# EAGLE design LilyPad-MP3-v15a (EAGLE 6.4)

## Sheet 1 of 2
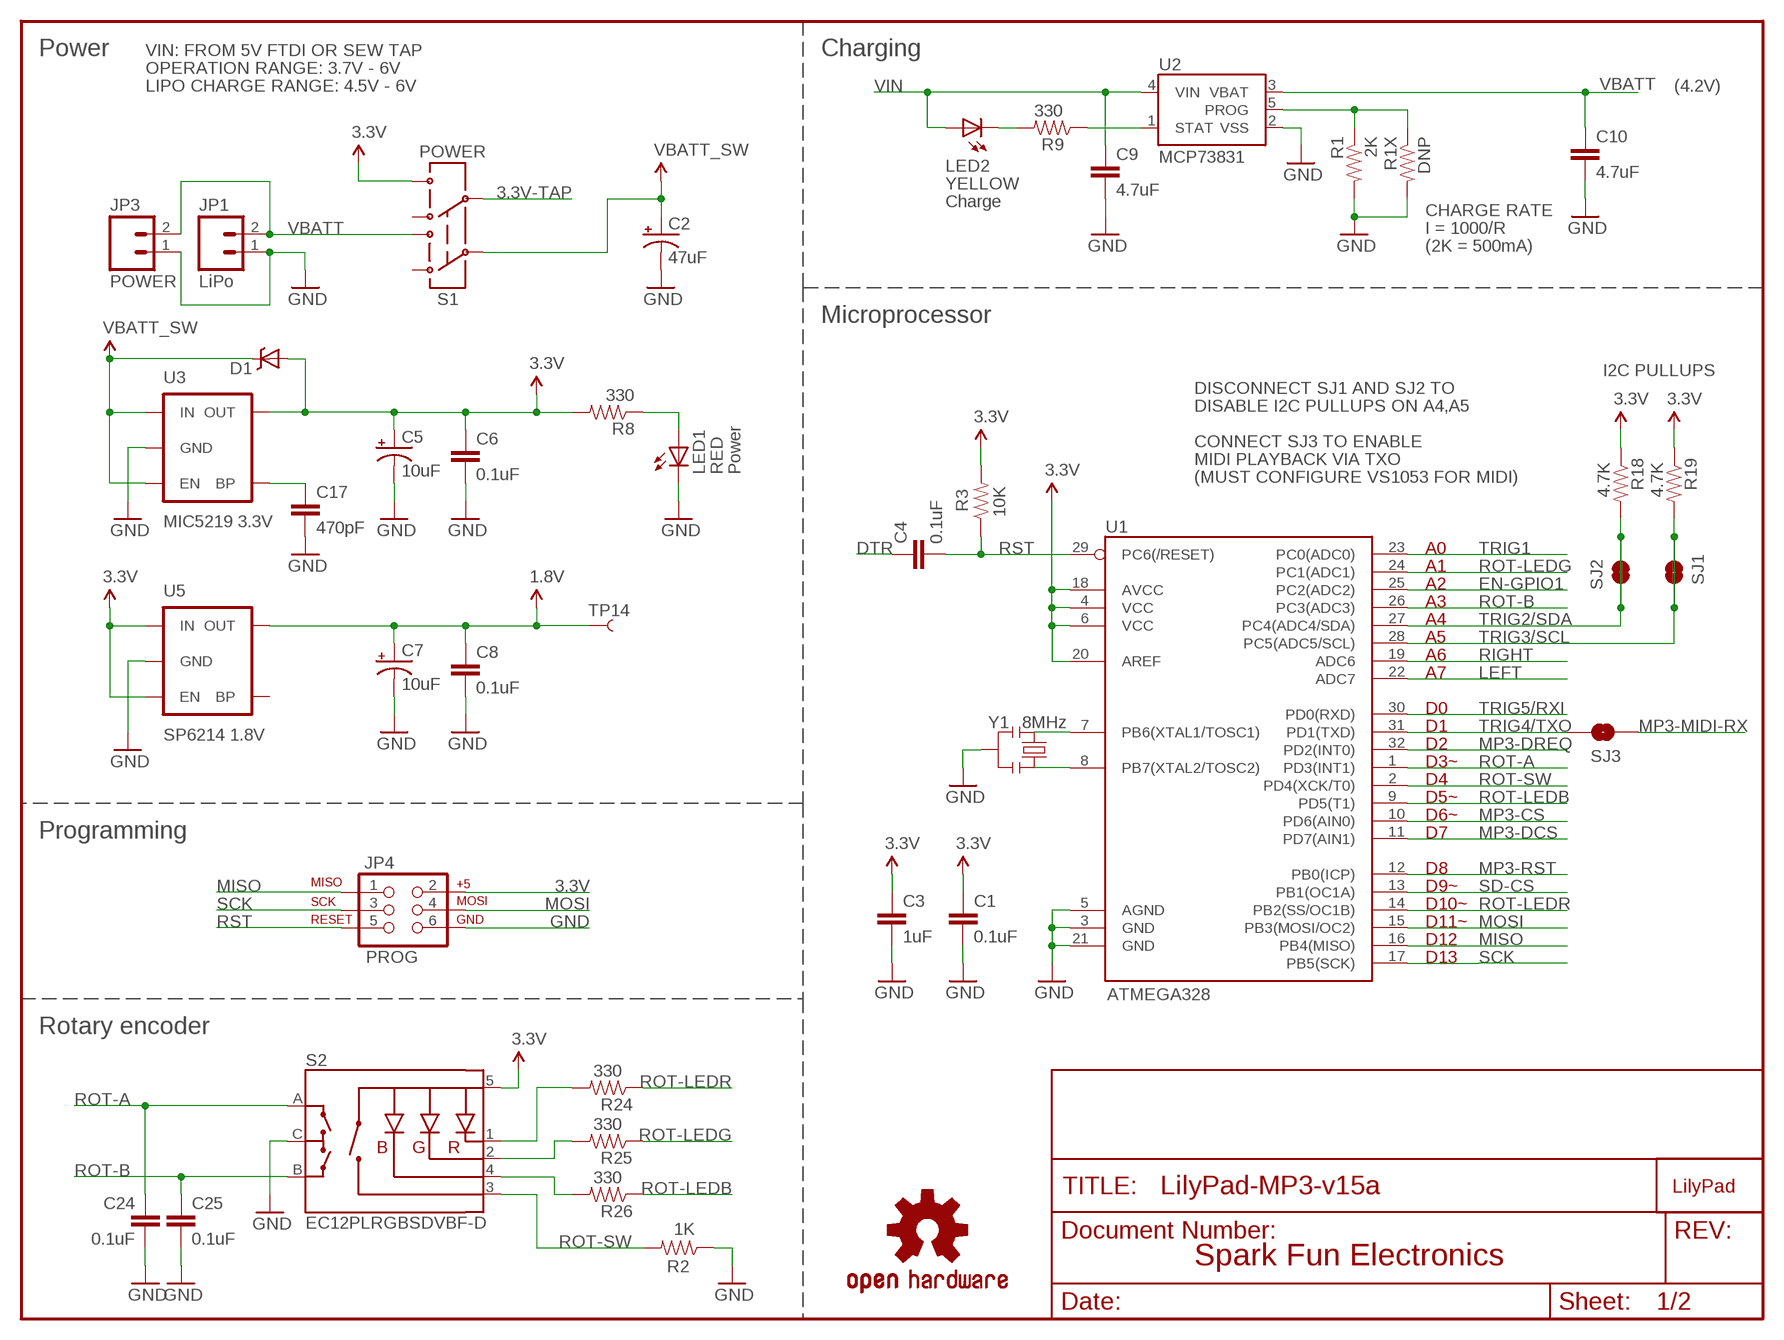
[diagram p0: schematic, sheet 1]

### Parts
C1  0.1uF  CAP0402-CAP  [0402-CAP]
C2  47uF  CAP_POL3528  [EIA3528]
C3  1uF  CAP0402-CAP  [0402-CAP]
C4  0.1uF  CAP0402-CAP  [0402-CAP]
C5  10uF  CAP_POL1206  [EIA3216]
C6  0.1uF  CAP0402-CAP  [0402-CAP]
C7  10uF  CAP_POL1206  [EIA3216]
C8  0.1uF  CAP0402-CAP  [0402-CAP]
C9  4.7uF  CAP0402-CAP  [0402-CAP]
C10  4.7uF  CAP0402-CAP  [0402-CAP]
C17  470pF  CAP0402-CAP  [0402-CAP]
C24  0.1uF  CAP0402-CAP  [0402-CAP]
C25  0.1uF  CAP0402-CAP  [0402-CAP]
D1  DIODE-SCHOTTKY  [SOD-523]
JP1  LiPo  M02-JST-2MM-SMT  [JST-2-SMD]
JP3  POWER  M02PTH  [1X02]
JP4  PROG  AVR_SPI_PRG_6NS  [2X3-NS]
LED1  RED  LED0603  [LED-0603]
LED2  YELLOW  LED0603  [LED-0603]
R1  2K  RESISTOR0402-RES  [0402-RES]
R1X  DNP  RESISTORAXIAL-0.3  [AXIAL-0.3]
R2  1K  RESISTOR0402-RES  [0402-RES]
R3  10K  RESISTOR0402-RES  [0402-RES]
R8  330  RESISTOR0402-RES  [0402-RES]
R9  330  RESISTOR0402-RES  [0402-RES]
R18  4.7K  RESISTOR0402-RES  [0402-RES]
R19  4.7K  RESISTOR0402-RES  [0402-RES]
R24  330  RESISTOR0402-RES  [0402-RES]
R25  330  RESISTOR0402-RES  [0402-RES]
R26  330  RESISTOR0402-RES  [0402-RES]
S1  POWER  AYZ0202  [AYZ0202]
S2  EC12PLRGBSDVBF-D  ENCODER_3LED_CA  [ENCODER_LED_3]
SJ1  SOLDERJUMPERNO  [SJ_2S-NO]
SJ2  SOLDERJUMPERNO  [SJ_2S-NO]
SJ3  SOLDERJUMPERNO  [SJ_2S-NO]
TP14  1.8V  TEST-POINT3X5  [PAD.03X.05]
U1  ATMEGA328  ATMEGA168  [TQFP32-08]
U2  MCP73831  [SOT23-5]
U3  MIC5219 3.3V  V_REG_LDOSMD  [SOT23-5]
U5  SP6214 1.8V  V_REG_LDOSMD2  [SC70]
U$1  LOGO-LPLP  [LOGO-LILYPAD]
U$4  OSHW-LOGOM  [OSHW-LOGO-M]
Y1  8MHz  RESONATORSMD  [RESONATOR-SMD]

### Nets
1.8V: C7.A(+) C8.1 TP14.P$1 U5.5(OUT) ; also sheet 2
3.3V: C1.1 C3.1 C5.A(+) C6.1 D1.A JP4.2 R3.2 R8.2 R18.1 R19.1 S1.4 S2.5(+) U1.4(VCC) U1.6(VCC) U1.18(AVCC) U1.20(AREF) U3.5(OUT) U5.1(IN) U5.3(EN) ; also sheet 2
3.3V-TAP: S1.5 ; also sheet 2
DTR: C4.1 ; also sheet 2
EN-GPIO1: U1.25(PC2(ADC2)) ; also sheet 2
GND [VCC]: C1.2 C2.C(-) C3.2 C5.C(-) C6.2 C7.C(-) C8.2 C9.2 C10.2 C17.2 C24.2 C25.2 JP1.1 JP3.1 JP4.6 LED1.C R1.2 R1X.P$2 R2.1 S2.C U1.3(GND) U1.5(AGND) U1.21(GND) U2.2(VSS) U3.2(GND) U5.2(GND) Y1.2 ; also sheet 2
LEFT: U1.22(ADC7) ; also sheet 2
MISO: JP4.1 U1.16(PB4(MISO)) ; also sheet 2
MOSI: JP4.4 U1.15(PB3(MOSI/OC2)) ; also sheet 2
MP3-CS: U1.10(PD6(AIN0)) ; also sheet 2
MP3-DCS: U1.11(PD7(AIN1)) ; also sheet 2
MP3-DREQ: U1.32(PD2(INT0)) ; also sheet 2
MP3-MIDI-RX: SJ3.1 ; also sheet 2
MP3-RST: U1.12(PB0(ICP)) ; also sheet 2
N$1: U1.7(PB6(XTAL1/TOSC1)) Y1.1
N$3: U1.8(PB7(XTAL2/TOSC2)) Y1.3
N$6: LED1.A R8.1
N$8: LED2.C R9.2
N$12: R24.2 S2.1(-R)
N$13: R25.2 S2.2(-G)
N$14: R26.2 S2.4(-B)
N$70: C17.1 U3.4(BP)
PROG: R1.1 R1X.P$1 U2.5(PROG)
RIGHT: U1.19(ADC6) ; also sheet 2
ROT-A: C24.1 S2.A U1.1(PD3(INT1))
ROT-B: C25.1 S2.B U1.26(PC3(ADC3))
ROT-LEDB: R26.1 U1.9(PD5(T1))
ROT-LEDG: R25.1 U1.24(PC1(ADC1))
ROT-LEDR: R24.1 U1.14(PB2(SS/OC1B))
ROT-SW: R2.2 S2.3(SW) U1.2(PD4(XCK/T0))
RST: C4.2 JP4.5 R3.1 U1.29(PC6(/RESET))
SCK: JP4.3 U1.17(PB5(SCK)) ; also sheet 2
SD-CS: U1.13(PB1(OC1A)) ; also sheet 2
STAT: R9.1 U2.1(STAT)
TRIG1: U1.23(PC0(ADC0)) ; also sheet 2
TRIG2/SDA: R18.2 SJ2.1 SJ2.2 U1.27(PC4(ADC4/SDA)) ; also sheet 2
TRIG3/SCL: R19.2 SJ1.1 SJ1.2 U1.28(PC5(ADC5/SCL)) ; also sheet 2
TRIG4/TXO: SJ3.2 U1.31(PD1(TXD)) ; also sheet 2
TRIG5/RXI: U1.30(PD0(RXD)) ; also sheet 2
VBATT: C10.1 JP1.2 JP3.2 S1.1 U2.3(VBAT)
VBATT_SW: C2.A(+) D1.C S1.2 U3.1(IN) U3.3(EN) ; also sheet 2
VIN: C9.1 LED2.A U2.4(VIN) ; also sheet 2
Unconnected: S1.3 S1.6 U5.4(BP)

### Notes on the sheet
- Power | VIN: FROM 5V FTDI OR SEW TAP | Charging
- OPERATION RANGE: 3.7V - 6V
- LIPO CHARGE RANGE: 4.5V - 6V | (4.2V)
- Charge
- CHARGE RATE
- I = 1000/R
- (2K = 500mA)
- Microprocessor
- I2C PULLUPS
- DISCONNECT SJ1 AND SJ2 TO
- DISABLE I2C PULLUPS ON A4,A5
- CONNECT SJ3 TO ENABLE
- MIDI PLAYBACK VIA TXO
- Power
- (MUST CONFIGURE VS1053 FOR MIDI)
- A0
- A1
- A2
- A3
- A4
- A5
- A6
- A7
- D0
- D1
- D2
- D3~
- D4
- D5~
- D6~
- Programming | D7
- D8
- D9~
- D10~
- D11~
- D12
- D13
- Rotary encoder
- Spark Fun Electronics

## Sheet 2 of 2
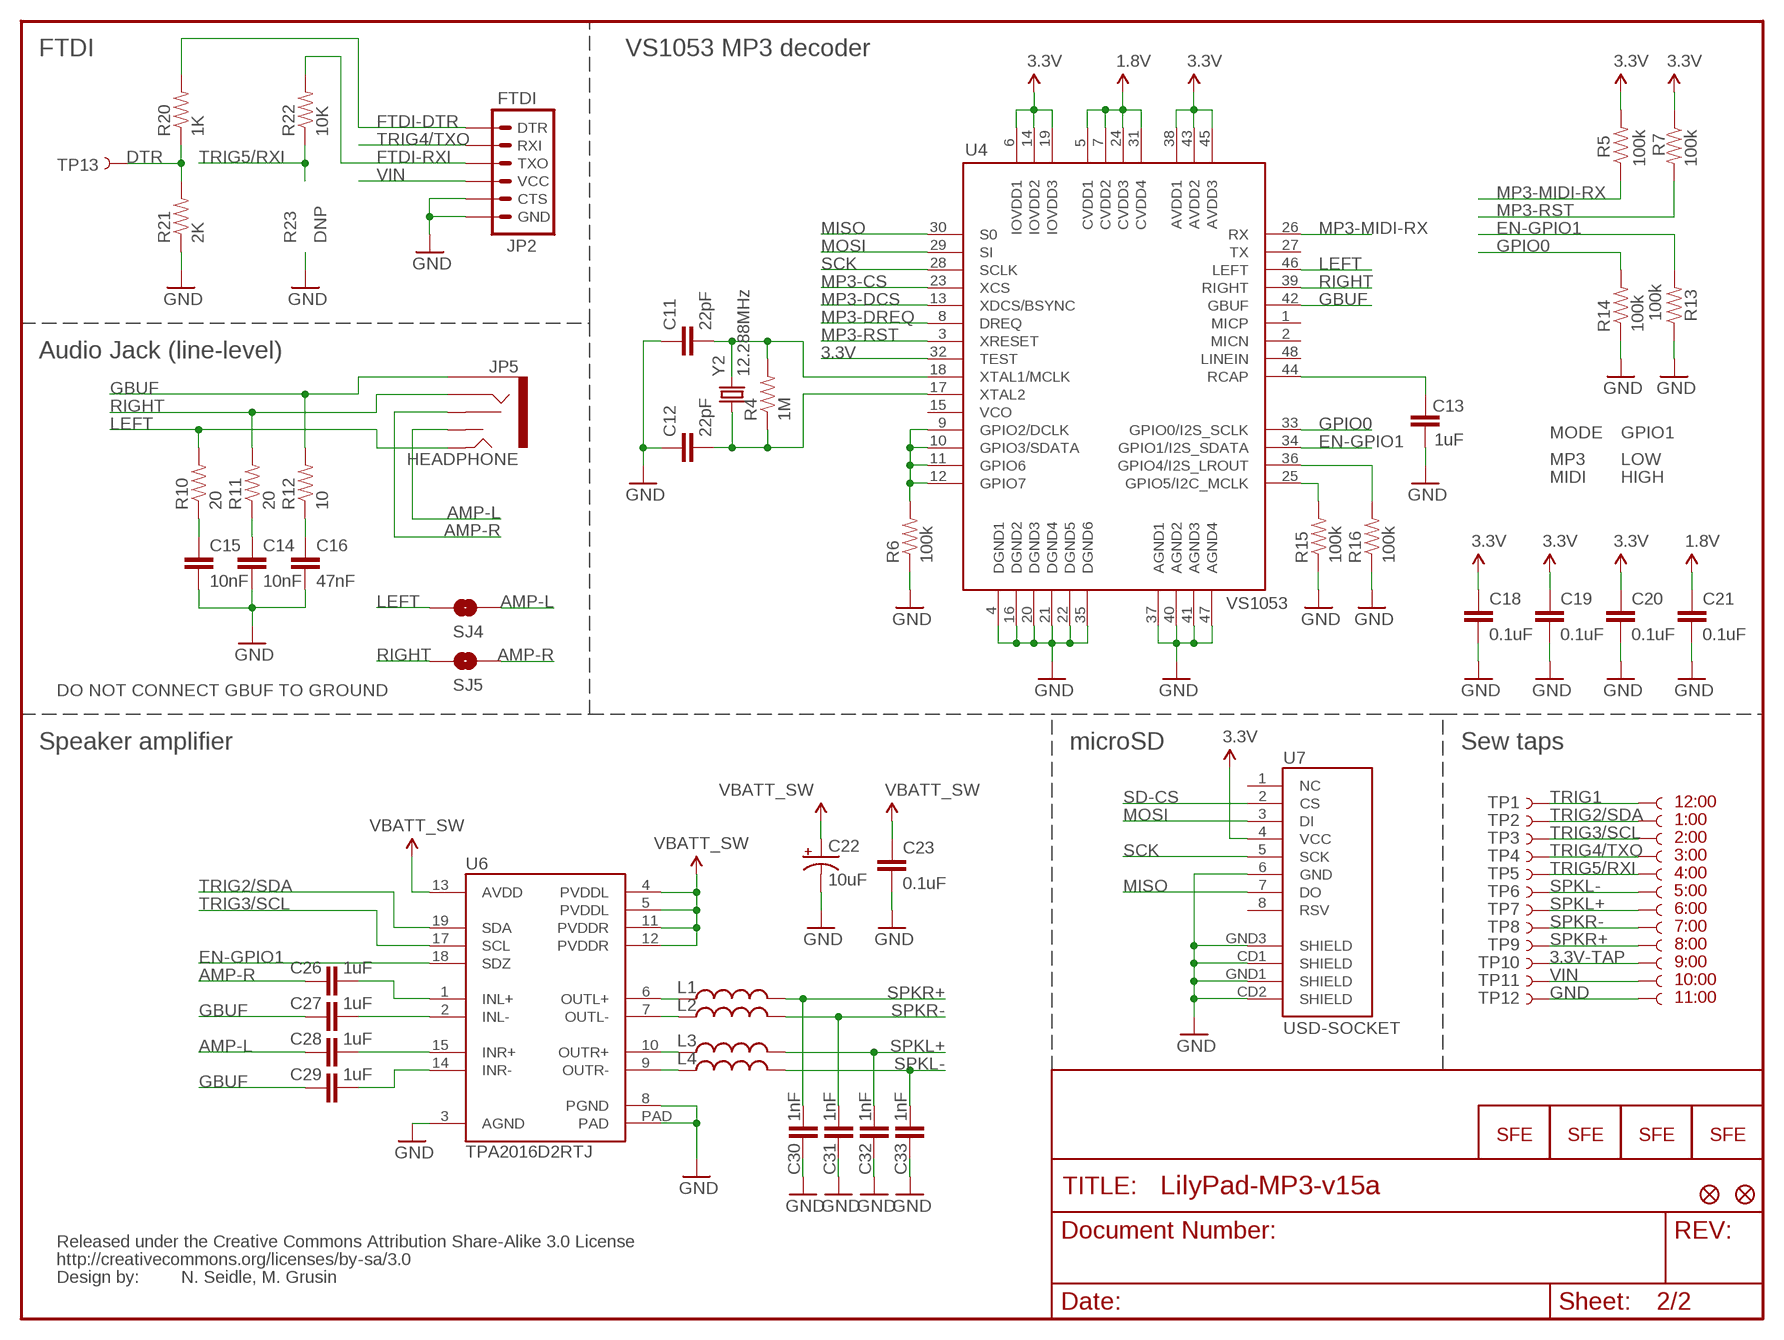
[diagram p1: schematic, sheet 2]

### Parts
C11  22pF  CAP0402-CAP  [0402-CAP]
C12  22pF  CAP0402-CAP  [0402-CAP]
C13  1uF  CAP0402-CAP  [0402-CAP]
C14  10nF  CAP0402-CAP  [0402-CAP]
C15  10nF  CAP0402-CAP  [0402-CAP]
C16  47nF  CAP0402-CAP  [0402-CAP]
C18  0.1uF  CAP0402-CAP  [0402-CAP]
C19  0.1uF  CAP0402-CAP  [0402-CAP]
C20  0.1uF  CAP0402-CAP  [0402-CAP]
C21  0.1uF  CAP0402-CAP  [0402-CAP]
C22  10uF  CAP_POL1206  [EIA3216]
C23  0.1uF  CAP0402-CAP  [0402-CAP]
C26  1uF  CAP0402-CAP  [0402-CAP]
C27  1uF  CAP0402-CAP  [0402-CAP]
C28  1uF  CAP0402-CAP  [0402-CAP]
C29  1uF  CAP0402-CAP  [0402-CAP]
C30  1nF  CAP0402-CAP  [0402-CAP]
C31  1nF  CAP0402-CAP  [0402-CAP]
C32  1nF  CAP0402-CAP  [0402-CAP]
C33  1nF  CAP0402-CAP  [0402-CAP]
JP2  FTDI  ARDUINO_SERIAL_PROGRAMSMD  [1X06-SMD]
JP5  HEADPHONE  AUDIO-JACK2SMD  [AUDIO-JACK-3.5MM-SMD]
JP6  LOGO-SFENW2  [SFE-NEW-WEB]
JP7  FIDUCIALUFIDUCIAL  [MICRO-FIDUCIAL]
JP8  FIDUCIALUFIDUCIAL  [MICRO-FIDUCIAL]
L1  INDUCTOR0805  [0805]
L2  INDUCTOR0805  [0805]
L3  INDUCTOR0805  [0805]
L4  INDUCTOR0805  [0805]
LOGO1  LOGO-SFESK  [SFE-LOGO-FLAME]
LOGO2  LOGO-SFENEW  [SFE-NEW-WEBLOGO]
LOGO3  LOGO-SFESK  [SFE-LOGO-FLAME]
R4  1M  RESISTOR0402-RES  [0402-RES]
R5  100k  RESISTOR0402-RES  [0402-RES]
R6  100k  RESISTOR0402-RES  [0402-RES]
R7  100k  RESISTOR0402-RES  [0402-RES]
R10  20  RESISTOR0402-RES  [0402-RES]
R11  20  RESISTOR0402-RES  [0402-RES]
R12  10  RESISTOR0402-RES  [0402-RES]
R13  100k  RESISTOR0402-RES  [0402-RES]
R14  100k  RESISTOR0402-RES  [0402-RES]
R15  100k  RESISTOR0402-RES  [0402-RES]
R16  100k  RESISTOR0402-RES  [0402-RES]
R20  1K  RESISTOR0402-RES  [0402-RES]
R21  2K  RESISTOR0402-RES  [0402-RES]
R22  10K  RESISTOR0402-RES  [0402-RES]
SJ4  SOLDERJUMPERNO  [SJ_2S-NO]
SJ5  SOLDERJUMPERNO  [SJ_2S-NO]
ST1  TRIG2/SDA  SEWTAP9  [PETAL-LONG-1-2SIDE]
ST2  TRIG3/SCL  SEWTAP9  [PETAL-LONG-1-2SIDE]
ST3  TRIG4/TXO  SEWTAP9  [PETAL-LONG-1-2SIDE]
ST4  TRIG5/RXI  SEWTAP9  [PETAL-LONG-1-2SIDE]
ST5  SPKL-  SEWTAP9  [PETAL-LONG-1-2SIDE]
ST6  SPKL+  SEWTAP9  [PETAL-LONG-1-2SIDE]
ST7  SPKR-  SEWTAP9  [PETAL-LONG-1-2SIDE]
ST8  SPKR+  SEWTAP9  [PETAL-LONG-1-2SIDE]
ST9  3.3V  SEWTAP9  [PETAL-LONG-1-2SIDE]
ST10  VIN  SEWTAP9  [PETAL-LONG-1-2SIDE]
ST11  GND  SEWTAP9  [PETAL-LONG-1-2SIDE]
ST12  TRIG1  SEWTAP9  [PETAL-LONG-1-2SIDE]
TP1  TRIG1  TEST-POINT-PTH-LARGE  [1X01NS]
TP2  TRIG2/SDA  TEST-POINT-PTH-LARGE  [1X01NS]
TP3  TRIG3/SCL  TEST-POINT-PTH-LARGE  [1X01NS]
TP4  TRIG4/TXO  TEST-POINT-PTH-LARGE  [1X01NS]
TP5  TRIG5/RXI  TEST-POINT-PTH-LARGE  [1X01NS]
TP6  SPKL-  TEST-POINT-PTH-LARGE  [1X01NS]
TP7  SPKL+  TEST-POINT-PTH-LARGE  [1X01NS]
TP8  SPKR-  TEST-POINT-PTH-LARGE  [1X01NS]
TP9  SPKR+  TEST-POINT-PTH-LARGE  [1X01NS]
TP10  3.3V  TEST-POINT-PTH-LARGE  [1X01NS]
TP11  VIN  TEST-POINT-PTH-LARGE  [1X01NS]
TP12  GND  TEST-POINT-PTH-LARGE  [1X01NS]
TP13  DTR  TEST-POINT3X5  [PAD.03X.05]
U4  VS1053  VS1033  [LQFP-48]
U6  TPA2016D2RTJ  [QFN-20-0.5MM]
U7  USD-SOCKET  USD-SOCKETNEW  [MICRO-SD-SOCKET-PP]
U$12  CREATIVE_COMMONS  [CREATIVE_COMMONS]
Y2  12.288MHz  CRYSTAL5X3  [CRYSTAL-SMD-5X3]

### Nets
1.8V: C21.1 U4.5(CVDD1) U4.7(CVDD2) U4.24(CVDD3) U4.31(CVDD4) ; also sheet 1
3.3V: C18.1 C19.1 C20.1 R5.2 R7.1 U4.6(IOVDD1) U4.14(IOVDD2) U4.19(IOVDD3) U4.32(TEST) U4.38(AVDD1) U4.43(AVDD2) U4.45(AVDD3) U7.4(VCC) ; also sheet 1
3.3V-TAP: ST9.1 TP10.1 ; also sheet 1
AMP-L: C28.1 JP5.TSH SJ4.1
AMP-LX: C26.2 U6.1(INL+)
AMP-R: C26.1 JP5.RSH SJ5.1
AMP-RX: C28.2 U6.15(INR+)
DTR: R20.1 R21.2 TP13.P$1 ; also sheet 1
EN-GPIO1: R13.2 U4.34(GPIO1/I2S_SDATA) U6.18(SDZ) ; also sheet 1
FTDI-DTR: JP2.1(DTR) R20.2
FTDI-RXI: JP2.3(TXO) R22.2
G1: R6.2 U4.9(GPIO2/DCLK) U4.10(GPIO3/SDATA) U4.11(GPIO6) U4.12(GPIO7)
G2: R15.2 U4.25(GPIO5/I2C_MCLK)
GBUF: C27.1 C29.1 JP5.SLEEVE R12.2 U4.42(GBUF)
GBUFLX: C27.2 U6.2(INL-)
GBUFRX: C29.2 U6.14(INR-)
GND [VCC]: C11.1 C12.1 C13.1 C14.2 C15.2 C16.2 C18.2 C19.2 C20.2 C21.2 C22.C(-) C23.2 C30.2 C31.2 C32.2 C33.2 JP2.5(CTS) JP2.6(GND) R6.1 R13.1 R14.1 R15.1 R16.1 R21.1 ST11.1 TP12.1 U4.4(DGND1) U4.16(DGND2) U4.20(DGND3) U4.21(DGND4) U4.22(DGND5) U4.35(DGND6) U4.37(AGND1) U4.40(AGND2) U4.41(AGND3) U4.47(AGND4) U6.3(AGND) U6.8(PGND) U6.PAD U7.6(GND) U7.CD1(SHIELD) U7.CD2(SHIELD) U7.GND1(SHIELD) U7.GND3(SHIELD) ; also sheet 1
GPIO0: R14.2 U4.33(GPIO0/I2S_SCLK)
LEFT: JP5.TIP R10.2 SJ4.2 U4.46(LEFT) ; also sheet 1
MISO: U4.30(S0) U7.7(DO) ; also sheet 1
MOSI: U4.29(SI) U7.3(DI) ; also sheet 1
MP3-CS: U4.23(XCS) ; also sheet 1
MP3-DCS: U4.13(XDCS/BSYNC) ; also sheet 1
MP3-DREQ: U4.8(DREQ) ; also sheet 1
MP3-MIDI-RX: R5.1 U4.26(RX) ; also sheet 1
MP3-RST: R7.2 U4.3(XRESET) ; also sheet 1
N$4: C13.2 U4.44(RCAP)
N$5: C16.1 R12.1
N$7: C15.1 R10.1
N$9: C11.2 R4.2 U4.18(XTAL1/MCLK) Y2.3
N$10: C12.2 R4.1 U4.17(XTAL2) Y2.1
N$11: C14.1 R11.1
N$16: L1.1 U6.6(OUTL+)
N$17: L2.1 U6.7(OUTL-)
N$18: L3.1 U6.10(OUTR+)
N$19: L4.1 U6.9(OUTR-)
N$73: R16.2 U4.36(GPIO4/I2S_LROUT)
RIGHT: JP5.RING R11.2 SJ5.2 U4.39(RIGHT) ; also sheet 1
SCK: U4.28(SCLK) U7.5(SCK) ; also sheet 1
SD-CS: U7.2(CS) ; also sheet 1
SPKL+: C32.1 L3.2 ST6.1 TP7.1
SPKL-: C33.1 L4.2 ST5.1 TP6.1
SPKR+: C30.1 L1.2 ST8.1 TP9.1
SPKR-: C31.1 L2.2 ST7.1 TP8.1
TRIG1: ST12.1 TP1.1 ; also sheet 1
TRIG2/SDA: ST1.1 TP2.1 U6.19(SDA) ; also sheet 1
TRIG3/SCL: ST2.1 TP3.1 U6.17(SCL) ; also sheet 1
TRIG4/TXO: JP2.2(RXI) ST3.1 TP4.1 ; also sheet 1
TRIG5/RXI: R22.1 ST4.1 TP5.1 ; also sheet 1
VBATT_SW: C22.A(+) C23.1 U6.4(PVDDL) U6.5(PVDDL) U6.11(PVDDR) U6.12(PVDDR) U6.13(AVDD) ; also sheet 1
VIN: JP2.4(VCC) ST10.1 TP11.1 ; also sheet 1
Unconnected: U4.1(MICP) U4.2(MICN) U4.15(VCO) U4.27(TX) U4.48(LINEIN) U7.1(NC) U7.8(RSV)

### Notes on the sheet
- FTDI | VS1053 MP3 decoder
- R23 | DNP
- Audio Jack (line-level)
- MODE | GPIO1
- MP3 | LOW
- MIDI | HIGH
- DO NOT CONNECT GBUF TO GROUND
- Speaker amplifier | microSD | Sew taps
- 12:00
- 1:00
- 2:00
- 3:00
- 4:00
- 5:00
- 6:00
- 7:00
- 8:00
- 9:00
- 10:00
- 11:00
- N. Seidle, M. Grusin

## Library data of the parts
C1 C3 C4 C6 C8-C21 C23-C29 = SparkFun:CAP: Capacitor
C2 C5 C7 C22 = SparkFun:CAP_POL: Capacitor Polarized
C30-C33 = SparkFun-Passives:CAP: Capacitor
D1 = SparkFun-DiscreteSemi:DIODE-SCHOTTKY: Commonly MBRA140.
JP1 JP3 = SparkFun:M02: Header 2
JP2 = SparkFun:ARDUINO_SERIAL_PROGRAM
JP4 = SparkFun:AVR_SPI_PRG_6: AVR ISP 6 Pin This is the reduced ISP connector for AVR programming. Common on Arduino. This footprint will take up less PCB space and can be used with a 10-pin to 6-pin adapter such as SKU: BOB-08508
JP5 = SparkFun:AUDIO-JACK2
JP6 LOGO1-LOGO3 = SparkFun:LOGO-SFE: Spark Fun Electronics PCB Logo
JP7 JP8 = SparkFun-Aesthetics:FIDUCIAL: Fiducial Alignment Points
L1-L4 = SparkFun-Passives:INDUCTOR: Inductors
LED1 LED2 = SparkFun:LED: LEDs
R1 R1X R2-R16 R18-R22 R24-R26 = SparkFun:RESISTOR: Resistor
S1 = SparkFun:AYZ0202: SPDT Slide Switch Simple SMD single-pull double-throw slide switch. Good for less than 350mA power switch, switching UARTs between devices, etc. Spark Fun Electronics SKU : COM-00597
S2 = mike-temp:ENCODER_3LED_CA
SJ1-SJ5 = SparkFun:SOLDERJUMPER: Solder Jumper
ST1-ST12 = LilyPad-Wearables:SEWTAP
TP1-TP12 = mike-temp:TEST-POINT
TP13 TP14 = SparkFun:TEST-POINT
U1 = SparkFun:ATMEGA168
U2 = SparkFun:MCP73831: Microchip's MCP73831 Miniature single cell, fully integrated Li-Ion, Li-polymer charge management controller http://ww1.microchip.com/downloads/en/DeviceDoc/21984a.pdf
U3 U5 = SparkFun:V_REG_LDO: Voltage Regulator LDO Standard 150mA LDO voltage regulator in SOT-23 layout. Micrel part MIC5205. BP (by-pass) pin is used to lower output noise with 470pF cap.
U4 = SparkFun:VS1033
U6 = mike-temp:TPA2016D2: 2.8-W/Ch Stereo Class-D Audio Amplifier with I2C volume control, DRC and AGC The TPA2016D2 is a stereo, filter-free Class-D audio power amplifier with volume control, dynamic range compression (DRC) and automatic gain control (AGC). It is available in a 2.2 mm x 2.2 mm WCSP package and 20-pin QFN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
U7 = SparkFun:USD-SOCKET: microSD Socket Push-push type uSD socket. Schematic element and footprint production proven. Spark Fun Electronics SKU : PRT-00127. tDoc lines correctly indicate media card edge positions when inserting (unlocked, locked, depressed).
U$1 = LilyPad-Wearables:LOGO-LP
U$4 = SparkFun:OSHW-LOGO: Open Source Hardware Logo This logo indicates the piece of hardware it is found on incorporates a OSHW license and/or adheres to the definition of open source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
U$12 = SparkFun:CREATIVE_COMMONS
Y1 = SparkFun:RESONATOR: Resonator Small SMD resonator. This is the itty bitty 10/20MHz resonators with built in caps. CSTCE10M0G55 and CSTCE20M0V53. Footprint has been reviewed closely but hasn't been tested yet.
Y2 = SparkFun:CRYSTAL: Crystals

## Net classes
0 default: clearance 0.254 mm
1 VCC: width 0.254 mm, clearance 0.254 mm

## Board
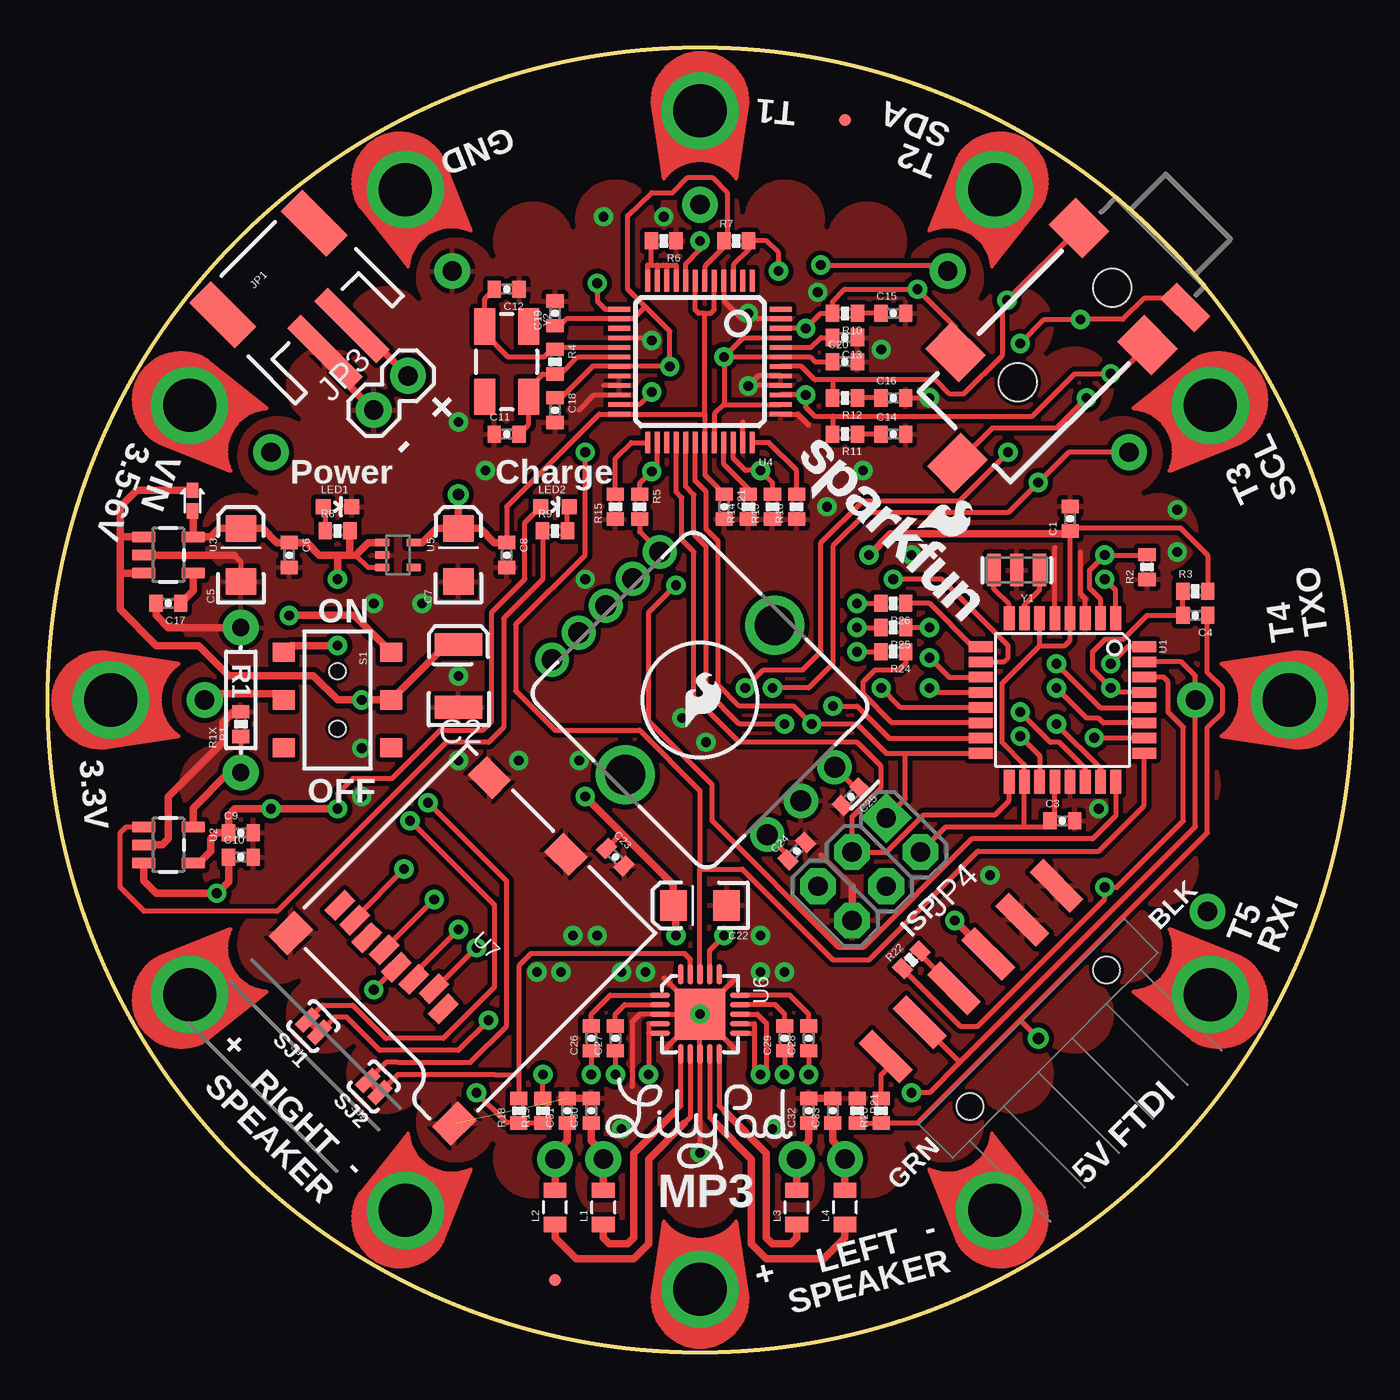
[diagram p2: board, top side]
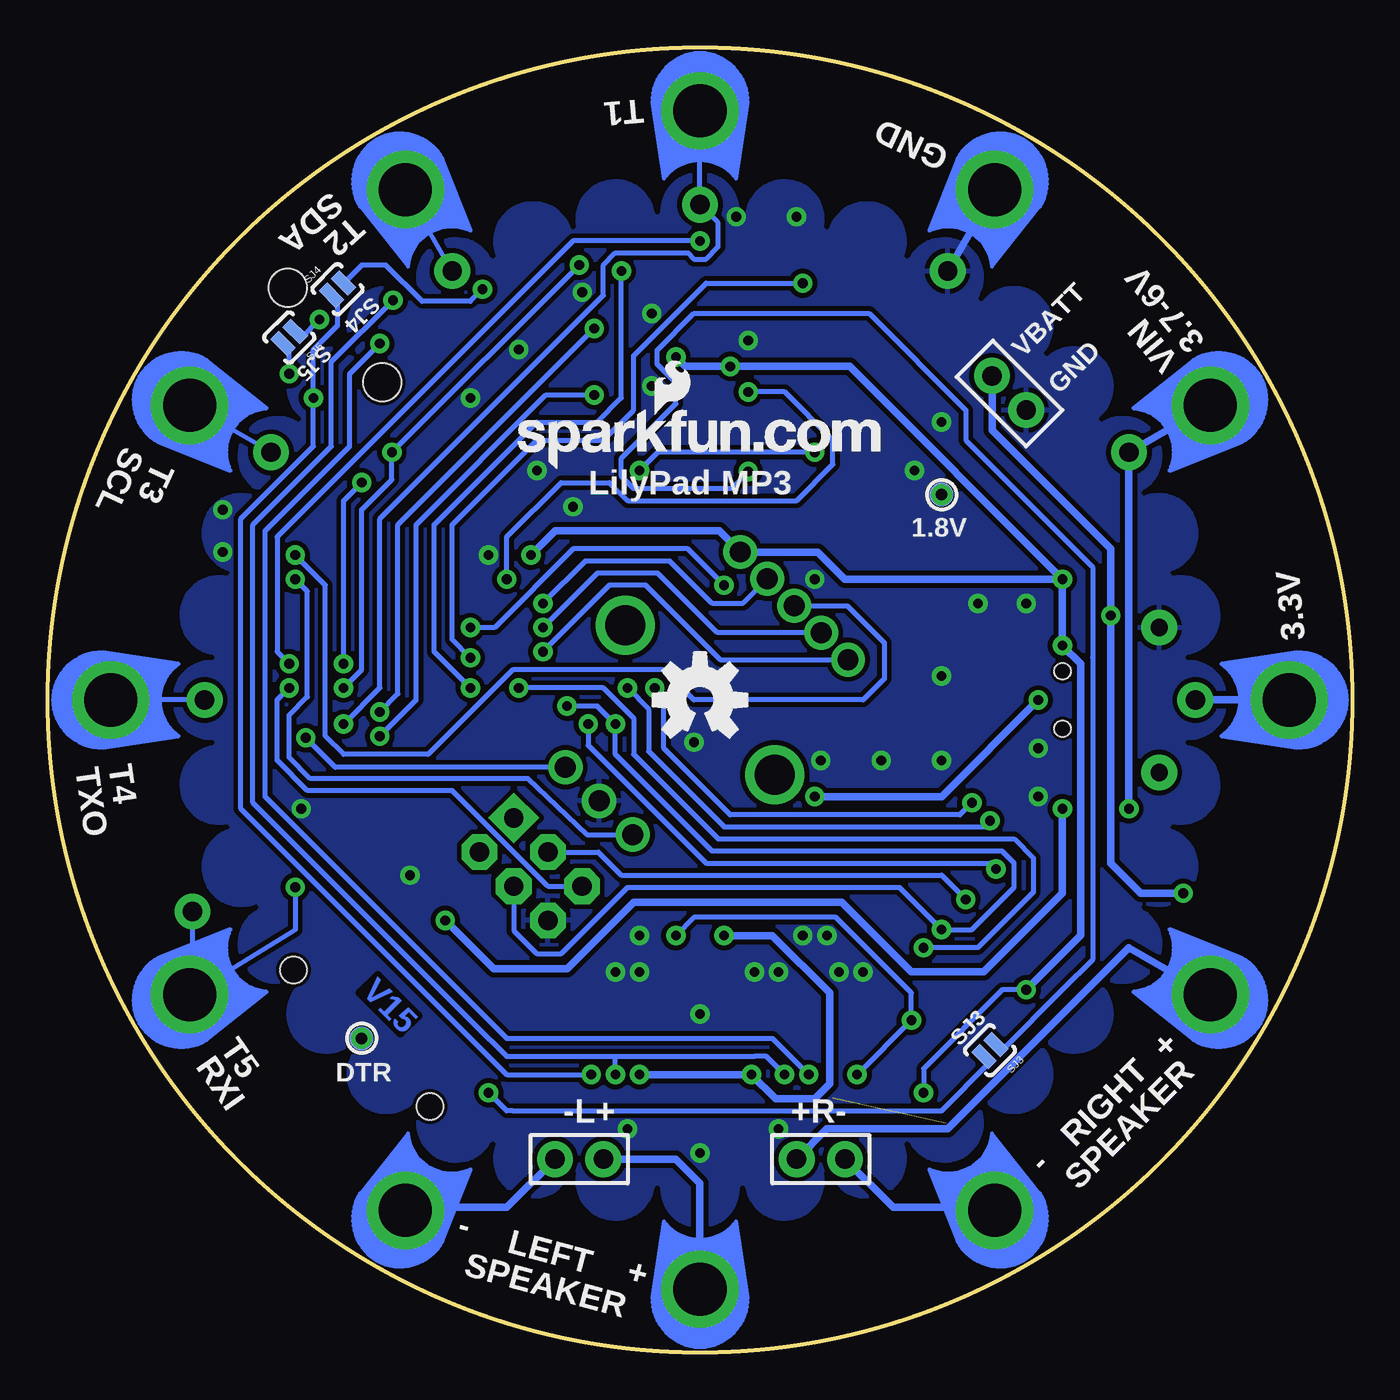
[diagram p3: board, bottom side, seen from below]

Size 68.58 x 68.58 mm. Coordinates in mm from the lower left corner, seen from the top.
Outline: circle at 34.29,34.29 radius 34.29
Copper layers (1*16): Top 0.035mm / dielectric 1.5mm / Bottom 0.035mm
Design rules: minimum track width 8mil, minimum drill 20mil, track to track 5mil, track to pad 5mil, pad to pad 5mil, via to via 5mil, smd to smd 5mil, copper to edge 8mil, drill to drill 8mil, minimum pad ring 12mil, minimum via ring 10mil, stop-mask expansion 4mil, vias tented up to drill 20mil, thermal gap 10mil
tRestrict: area 3.1,3.1 to 65.5,65.5; area 59.9,31.8 to 63.3,36.8; area 59.2,36.5 to 63.3,41.8; area 57.6,41 to 62.4,46.6; area 55.4,45.2 to 60.7,51; area 52.5,49.1 to 58.1,54.9; area 49.1,52.5 to 54.9,58.1; area 45.2,55.4 to 51,60.7; area 41,57.6 to 46.6,62.4; area 36.5,59.2 to 41.8,63.3; area 31.8,59.9 to 36.8,63.3; area 26.8,59.2 to 32,63.3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
bRestrict: area 3.1,3.1 to 65.5,65.5; area 59.9,31.8 to 63.3,36.8; area 59.2,36.5 to 63.3,41.8; area 57.6,41 to 62.4,46.6; area 55.4,45.2 to 60.7,51; area 52.5,49.1 to 58.1,54.9; area 49.1,52.5 to 54.9,58.1; area 45.2,55.4 to 51,60.7; area 41,57.6 to 46.6,62.4; area 36.5,59.2 to 41.8,63.3; area 31.8,59.9 to 36.8,63.3; area 26.8,59.2 to 32,63.3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

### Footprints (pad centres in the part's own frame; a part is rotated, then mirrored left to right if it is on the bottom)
0402-CAP = smd 0.7 x 0.9: 1 -0.65,0; 2 0.65,0
EIA3528 = smd 1.2 x 2.5: A 1.65,0; C -1.65,0
EIA3216 = smd 1.4 x 1.6: A 1.4,0; C -1.4,0
SOD-523 = smd 0.8 x 0.6: A -0.55,0; C 0.55,0
JST-2-SMD = smd 1 x 4.6: 1 -1,-3.7; 2 1,-3.7 | smd 1.6 x 3.4: NC1 -3.4,1.5; NC2 3.4,1.5
1X06-SMD = smd 1 x 3: 1 -6.35,5; 2 -3.81,5; 3 -1.27,5; 4 1.27,5; 5 3.81,5; 6 6.35,5 | hole 1.4: -5.08,0; 5.08,0
1X02 = drill 1.016 pad 1.88: 1 0,0; 2 2.54,0
2X3-NS = drill 1.016 pad 1.88 square: 1 -2.54,-1.27 | drill 1.016 pad 1.88 octagon: 2 -2.54,1.27; 3 0,-1.27; 4 0,1.27; 5 2.54,-1.27; 6 2.54,1.27
AUDIO-JACK-3.5MM-SMD = smd 2 x 2.5: RING 4.3,3.45; SLEEVE 2.5,-3.45; TIP 11.7,-3.45 | smd 1.2 x 2.5: RSH 1.5,3.45 | smd 2.5 x 2: TSH 15.75,0.75 | hole 2: 3.5,0; 10.5,0
MICRO-FIDUCIAL = smd 0.635 x 0.635: 1 0,0
0805 = smd 0.8 x 1.2: 1 -0.9,0; 2 0.9,0
LED-0603 = smd 0.8 x 0.8: A 0,-0.75; C 0,0.75
0402-RES = smd 0.7 x 0.9: 1 -0.65,0; 2 0.65,0
AXIAL-0.3 = drill 0.9 pad 1.88: P$1 -3.81,0; P$2 3.81,0
AYZ0202 = smd 1 x 1.15: 1 -2.5,2.825; 2 0,2.825; 3 2.5,2.825; 4 -2.5,-2.825; 5 0,-2.825; 6 2.5,-2.825 | hole 0.85: 1.5,0; -1.5,0
ENCODER_LED_3 = drill 1.1 pad 1.778: 1 -4,7; 2 -2,7; 3 0,7; 4 2,7; 5 4,7 | drill 1.1 pad 1.8: A -2.5,-7.5; B 2.5,-7.5; C 0,-7.5 | drill 2.1: M1 -5.55,0; M2 5.55,0
SJ_2S-NO = smd 0.635 x 1.27: 1 -0.45,0; 2 0.45,0
PETAL-LONG-1-2SIDE = drill 2.794 pad 4.064: 1 0.03,0
1X01NS = drill 1.016 pad 1.88: 1 0,0
PAD.03X.05 = smd 1.27 x 1.27: P$1 0,0
TQFP32-08 = smd 1.27 x 0.559: 1 -4.293,2.8; 2 -4.293,2; 3 -4.293,1.2; 4 -4.293,0.4; 5 -4.293,-0.4; 6 -4.293,-1.2; 7 -4.293,-2; 8 -4.293,-2.8; 17 4.293,-2.8; 18 4.293,-2; 19 4.293,-1.2; 20 4.293,-0.4; 21 4.293,0.4; 22 4.293,1.2; 23 4.293,2; 24 4.293,2.8 | smd 0.559 x 1.27: 9 -2.8,-4.293; 10 -2,-4.293; 11 -1.2,-4.293; 12 -0.4,-4.293; 13 0.4,-4.293; 14 1.2,-4.293; 15 2,-4.293; 16 2.8,-4.293; 25 2.8,4.293; 26 2,4.293; 27 1.2,4.293; 28 0.4,4.293; 29 -0.4,4.293; 30 -1.2,4.293; 31 -2,4.293; 32 -2.8,4.293
SOT23-5 = smd 0.55 x 1.2: 1 -0.95,-1.3; 2 0,-1.3; 3 0.95,-1.3; 4 0.95,1.3; 5 -0.95,1.3
LQFP-48 = smd 0.254 x 1.143: 1 -2.75,-4.25; 2 -2.25,-4.25; 3 -1.75,-4.25; 4 -1.25,-4.25; 5 -0.75,-4.25; 6 -0.25,-4.25; 7 0.25,-4.25; 8 0.75,-4.25; 9 1.25,-4.25; 10 1.75,-4.25; 11 2.25,-4.25; 12 2.75,-4.25; 25 2.75,4.25; 26 2.25,4.25; 27 1.75,4.25; 28 1.25,4.25; 29 0.75,4.25; 30 0.25,4.25; 31 -0.25,4.25; 32 -0.75,4.25; 33 -1.25,4.25; 34 -1.75,4.25; 35 -2.25,4.25; 36 -2.75,4.25 | smd 1.143 x 0.254: 13 4.25,-2.75; 14 4.25,-2.25; 15 4.25,-1.75; 16 4.25,-1.25; 17 4.25,-0.75; 18 4.25,-0.25; 19 4.25,0.25; 20 4.25,0.75; 21 4.25,1.25; 22 4.25,1.75; 23 4.25,2.25; 24 4.25,2.75; 37 -4.25,2.75; 38 -4.25,2.25; 39 -4.25,1.75; 40 -4.25,1.25; 41 -4.25,0.75; 42 -4.25,0.25; 43 -4.25,-0.25; 44 -4.25,-0.75; 45 -4.25,-1.25; 46 -4.25,-1.75; 47 -4.25,-2.25; 48 -4.25,-2.75
SC70 = smd 0.4 x 0.75: 1 -0.65,-0.825; 2 0,-0.825; 3 0.65,-0.825; 4 0.65,0.825; 5 -0.65,0.825
QFN-20-0.5MM = smd 0.28 x 1.05: 1 -1,-2.1; 2 -0.5,-2.1; 3 0,-2.1; 4 0.5,-2.1; 5 1,-2.1; 11 1,2.1; 12 0.5,2.1; 13 0,2.1; 14 -0.5,2.1; 15 -1,2.1 | smd 1.05 x 0.28: 6 2.1,-1; 7 2.1,-0.5; 8 2.1,0; 9 2.1,0.5; 10 2.1,1; 16 -2.1,1; 17 -2.1,0.5; 18 -2.1,0; 19 -2.1,-0.5; 20 -2.1,-1 | smd 2.7 x 2.7: PAD 0,0
MICRO-SD-SOCKET-PP = smd 0.8 x 1.5: 1 -8.94,10.7; 2 -7.84,10.3; 3 -6.74,10.7; 4 -5.64,10.9; 5 -4.54,10.7; 6 -3.44,10.9; 7 -2.34,10.7; 8 -1.24,10.7 | smd 1.8 x 1.4: CD1 -2.05,0.4; CD2 -7.75,0.4 | smd 1.4 x 1.9: GND1 -13.6,14.55; GND3 -0.45,13.55
RESONATOR-SMD = smd 0.7 x 1.7: 1 -1.2,0; 2 0,0; 3 1.2,0
CRYSTAL-SMD-5X3 = smd 1.9 x 1.1: 1 -1.85,-1.15; 2 1.85,-1.15; 3 1.85,1.15; 4 -1.85,1.15

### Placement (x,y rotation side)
C1  53.74,43.81 90 top
C2  21.59,35.56 90 top
C3  53.34,27.94 0 top
C4  60.33,38.73 180 top
C5  10.16,41.91 90 top
C6  12.7,41.91 270 top
C7  21.59,41.91 90 top
C8  24.13,41.91 270 top
C9  10.16,27.3 0 top
C10  10.16,26.03 0 top
C11  24.13,48.26 0 top
C12  24.13,55.88 180 top
C13  41.91,53.34 180 top
C14  44.45,48.26 0 top
C15  44.45,54.61 0 top
C16  44.45,50.16 0 top
C17  6.35,39.37 180 top
C18  26.67,49.53 270 top
C19  26.67,54.61 90 top
C20  41.91,52.07 0 top
C21  35.56,44.45 270 top
C22  34.29,23.49 180 top
C23  29.84,26.03 315 top
C24  39.37,26.35 45 top
C25  42.23,29.21 225 top
C26  28.57,16.51 90 top
C27  29.84,16.51 90 top
C28  40,16.51 90 top
C29  38.73,16.51 90 top
C30  28.57,12.7 90 top
C31  27.3,12.7 90 top
C32  40,12.7 90 top
C33  41.27,12.7 90 top
D1  7.62,44.77 90 top
JP1  12.67,55.88 45 top
JP2  52.07,16.51 45 top
JP3  17.14,49.53 45 top
JP4  43.18,25.4 225 top
JP5  58.42,58.42 225 top
JP6  38.73,46.35 315 top
JP7  26.67,3.81 0 top
JP8  41.91,64.77 0 top
L1  29.21,7.62 90 top
L2  26.67,7.62 90 top
L3  39.37,7.62 90 top
L4  41.91,7.62 90 top
LED1  15.24,44.45 270 top
LED2  26.67,44.45 270 top
LOGO1  33.53,32.89 0 top
LOGO2  43.88,46.42 0 bottom
LOGO3  45.72,43.34 315 top
R1  10.16,33.02 90 top
R1X  10.16,34.29 90 top
R2  57.78,41.27 90 top
R3  60.33,40 0 top
R4  26.67,52.07 270 top
R5  31.11,44.45 270 top
R6  32.38,58.42 180 top
R7  36.2,58.42 0 top
R8  15.24,43.18 0 top
R9  26.67,43.18 0 top
R10  41.91,54.61 180 top
R11  41.91,48.26 180 top
R12  41.91,50.16 180 top
R13  38.1,44.45 90 top
R14  36.83,44.45 90 top
R15  29.84,44.45 90 top
R16  39.37,44.45 90 top
R18  24.77,12.7 90 top
R19  26.03,12.7 90 top
R20  43.81,12.7 90 top
R21  42.55,12.7 270 top
R22  45.4,20.64 45 top
R24  44.45,36.83 180 top
R25  44.45,38.1 180 top
R26  44.45,39.37 180 top
S1  15.24,34.29 270 top
S2  34.29,34.29 45 top
SJ1  13.97,17.14 135 top
SJ2  17.14,13.97 135 top
SJ3  19.05,15.88 225 bottom
SJ4  53.34,55.88 45 bottom
SJ5  55.88,53.34 225 bottom
ST1  49.79,61.14 240 top
ST2  61.14,49.79 210 top
ST3  65.29,34.29 180 top
ST4  61.14,18.79 150 top
ST5  49.79,7.44 120 top
ST6  34.29,3.29 90 top
ST7  18.79,7.44 60 top
ST8  7.44,18.79 30 top
ST9  3.29,34.29 0 top
ST10  7.44,49.79 330 top
ST11  18.79,61.14 300 top
ST12  34.29,65.29 270 top
TP1  34.29,60.33 0 top
TP2  47.31,56.83 0 top
TP3  56.83,47.31 0 top
TP4  60.33,34.29 0 top
TP5  60.96,23.18 0 top
TP6  41.91,10.16 0 top
TP7  39.37,10.16 0 top
TP8  26.67,10.16 0 top
TP9  29.21,10.16 0 top
TP10  8.25,34.29 0 top
TP11  11.75,47.31 0 top
TP12  21.27,56.83 0 top
TP13  52.07,16.51 0 bottom
TP14  21.59,45.09 0 bottom
U1  53.34,34.29 270 top
U2  6.35,26.67 270 top
U3  6.35,41.91 270 top
U4  34.29,52.07 180 top
U5  18.41,41.91 270 top
U6  34.29,17.78 270 top
U7  22.05,31.94 135 top
U$1  34.29,12.35 0 top
U$4  34.29,34.29 0 bottom
U$12  not placed on the board
Y1  50.94,41.12 180 top
Y2  24.13,52.07 270 top

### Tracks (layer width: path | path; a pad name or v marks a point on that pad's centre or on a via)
1.8V  (via drill 0.6)
  Top 0.254: C8.1 24.13,44.45 29,49.32 U4.24 34.54,49.32 | 34.54,49.32 U4.31 34.54,46.12 C21.1 | 34.54,54.61 34.22,54.61 34.04,54.79 U4.7 | 34.54,49.32 34.54,54.61 | 34.54,54.61 34.84,54.61 35.04,54.81 U4.5
  Top 0.406: U5.5 19.7,42.56 20.45,43.31 C7.A | C7.A 22.73,43.31 23.48,42.56 C8.1 | C7.A TP14.P$1
  other vias: 21.59,45.09
3.3V  (via drill 0.51)
  Top 0.254: U5.3 16.84,41.26 16.19,41.91 | v35.56,52.32 U4.43 40.07,52.32 40.32,52.07 C20.1 | 35.56,49.82 U4.38 | v35.56,52.32 35.56,49.82 | 35.56,49.82 35.53,49.82 35.04,49.33 U4.32 | 31.41,54.95 30.48,55.88 30.48,59.74 31.75,60.96 32.86,60.96 33.66,61.75 34.92,61.75 35.72,60.96 35.72,58.66 35.56,58.5 35.56,58.44 R7.1 35.55,58.09 34.54,57.08 U4.6 | U4.45 36.56,53.32 v35.56,52.32 | 31.41,54.95 32.7,53.66 v32.7,51.82 U4.19 28.64,51.82 27,50.18 C18.1 | 52.14,37.15 U1.6 | 52.14,37.15 53.45,37.15 53.74,37.44 U1.4 C1.1 53.74,43.26 53.82,43.34 59.53,43.34 60.97,41.89 R3.2 | v17.14,19.06 U7.4 | 51.34,27.62 47.2,27.62 JP4.2 | 51.34,27.62 U1.18 51.34,30.89 50.16,32.07 50.16,35.17 52.14,37.15 | 51.34,27.62 52.37,27.62 C3.1 52.94,28.19 U1.20 | C19.1 26.91,53.96 27.27,54.32 U4.14 30.77,54.32 31.41,54.95 | R19.1 R18.1 24.77,12.06 24.13,12.06 v22.54,13.65 | R5.2 31.11,43.12 S2.5
  Top 0.406: 15.24,41.91 14.29,41.91 13.64,42.56 C6.1 12.05,42.56 11.3,43.31 C5.A 9.02,43.31 8.57,42.86 U3.5 7.65,44.19 D1.A | U5.1 16.84,42.56 16.19,41.91 15.89,41.91 | 15.24,41.91 15.89,41.91 | v15.24,40.64 15.24,41.91 | C1.1 53.74,43.1 53.66,43.02 44.29,43.02 v43.18,41.91 | 15.89,41.91 R8.2 | S1.4 12.77,37.15 v15.24,37.15
  Bottom 0.254: v17.14,19.06 18.41,19.06 22.54,14.92 v22.54,13.65
  Bottom 0.406: v15.24,40.64 26.42,51.82 v32.7,51.82 35.06,51.82 v35.56,52.32 | v17.14,19.06 v17.14,19.05 16.51,19.68 14.29,21.92 14.29,36.2 v15.24,37.15 v15.24,40.64 | v15.24,40.64 26.67,40.64 28.1,42.07 S2.5 33.28,43.18 41.91,43.18 v43.18,41.91
3.3V-TAP
  Top 0.406: TP10.1 8.57,34.61 12.1,34.61 S1.5
  Bottom 0.406: ST9.1 TP10.1
AMP-L  (via drill 0.51)
  Top 0.254: JP5.TSH 49.64,48.58 53.02,48.58 v54.61,50.16 | C28.1 v40,14.61
  Bottom 0.254: SJ4.1 53.34,55.24 53.34,53.97 54.61,52.7 v54.61,50.16 54.61,47.62 58.42,43.81 58.42,28.57 46.35,16.51 44.45,14.61 v40,14.61
AMP-LX
  Top 0.254: C26.2 28.57,17.78 29.56,18.78 U6.1
AMP-R  (via drill 0.51)
  Top 0.254: v51.12,53.02 52.39,54.29 v54.29,54.29 56.52,54.29 57.63,55.4 59.31,55.4 JP5.RSH | C26.1 v28.57,14.61
  Bottom 0.254: v51.12,53.02 52.7,51.44 52.7,47.62 57.15,43.18 57.15,29.21 44.45,16.51 30.48,16.51 v28.57,14.61 | v54.29,54.29 55.24,53.34 SJ5.1
AMP-RX
  Top 0.254: C28.2 40,17.78 39.02,18.78 U6.15
DTR  (via drill 0.6)
  Top 0.254: 51.12,17.46 46.99,13.34 46.34,12.68 45.7,12.05 R20.1 R21.2 | 51.12,17.46 60.96,27.3 60.96,32.86 61.75,33.66 61.75,34.92 60.96,35.72 60.96,38.72 C4.1 | TP13.P$1 51.12,17.46
  other vias: 52.07,16.51
EN-GPIO1  (via drill 0.51)
  Top 0.254: U1.25 57.63,28.74 55.24,26.35 48.89,26.35 43.18,20.64 41.27,20.64 36.51,25.4 34.29,25.4 | v28.26,47.31 28.26,46.35 28.26,41.91 24.61,38.26 24.61,34.77 26.67,32.7 31.11,32.7 34.29,29.53 34.29,25.4 | R13.2 38.1,45.72 v37.46,46.35 36.67,46.35 36.04,46.99 U4.34 | U6.18 34.29,25.4
  Bottom 0.254: v28.26,47.31 28.57,47.31 36.51,47.31 v37.46,46.35
FTDI-DTR
  Top 0.254: R20.2 43.81,14.61 44.13,14.92 44.13,15.47 JP2.1
FTDI-RXI
  Top 0.254: JP2.3 45.86,20.92 R22.2
G1
  Top 0.254: U4.12 31.54,57.15 31.75,57.15 | 32.04,57.15 U4.11 | 31.75,57.15 32.04,57.15 | 32.54,57.15 U4.10 | 32.54,57.15 33.02,57.15 33.04,57.15 U4.9 | 32.04,57.15 32.54,57.15 | 31.75,57.15 32.37,57.15 | 31.75,57.15 32.05,57.15 | R6.2 31.73,57.15 31.75,57.15
G2
  Top 0.254: U4.25 30.67,47.82 29.84,46.99 R15.2
GBUF  (via drill 0.51)
  Top 0.254: U4.42 39.62,51.82 40.32,51.12 41.26,51.12 | 41.26,51.12 46.67,51.12 47.43,50.36 48.14,50.36 50.16,52.39 50.16,55.04 v50.42,55.3 JP5.SLEEVE | 41.26,51.12 R12.2 | C27.1 v29.84,14.61 | C29.1 v38.73,14.61
  Bottom 0.254: v50.42,55.3 53.66,52.07 53.66,47.62 57.78,43.5 57.78,28.89 46.2,17.3 44.45,15.56 38.73,15.56 | 38.73,15.56 31.43,15.56 30.8,15.56 v29.84,14.61 | v38.73,14.61 38.73,15.56
GBUFLX
  Top 0.254: C27.2 29.84,17.78 30.33,18.28 U6.2
GBUFRX
  Top 0.254: C29.2 38.73,17.78 38.25,18.28 U6.14
GND  (via drill 0.51)  (1 unrouted)
  Top 0.254: U4.16 31.77,53.32 v31.75,53.18 | U4.22 28.73,50.32 27.94,49.53 | U4.21 29.23,50.82 | C16.2 45.09,50.18 45.09,50.16 v46.35,50.16 | 14.58,52.1 JP1.1 | 9.8,41.91 10.16,41.55 C5.C | U4.35 36.54,48.89 | 42.28,24.5 40.64,26.14 | 30.72,13.97 30.72,17.38 31.11,17.78 U6.3 U6.PAD | U6.PAD 36.2,19.68 | U6.PAD 32.38,19.68 | U6.PAD 32.38,15.88 | U6.PAD 36.2,15.88 | v34.29,10.48 U6.8 U6.PAD | U4.4 35.54,55.27 36.51,54.29 v36.83,54.61 37.33,54.32 U4.47 | U4.40 36.85,50.82 v36.83,50.8 37.35,51.32 U4.41 | U4.37 39.42,49.32 40,48.74 | U1.3 54.54,39.6 54.29,39.85 54.29,42.07 | U1.5 52.94,42.31
  Top 0.406: C17.2 5.7,38.75 6.35,38.1 R1X.P$2 | U2.2 6.03,26.67 6.35,26.99 6.35,29.21 8.25,31.11 9.21,32.07 9.21,33.09 9.79,33.67 R1.2 | JP3.1 14.58,52.1 | 9.8,41.91 U3.2 | 42.28,24.5 JP4.6 | C31.2 C30.2 | C33.2 C32.2
  Bottom 0.406: TP12.1 ST11.1
  other vias: 32.38,59.69 43.81,52.7 16.51,29.21 49.53,25.08 55.24,28.57 34.61,32.07 23.02,46.35 26.99,20 40.48,55.72 29.21,59.69 17.14,39.37 31.43,20 21.59,48.89 34.29,17.78 28.26,40.64 37.46,20 45.4,41.91 30.16,11.75 38.1,11.75 38.73,20 24.77,31.11 21.59,31.11 40.96,44.45 28.89,21.91 27.62,21.91 25.72,20 27.94,31.11 21.59,35.56 59.37,42.07 59.37,44.29 42.86,46.35 33.34,33.34 16.51,31.75 37.46,21.91 19.68,39.37 30.16,20
  pour Top: 34.29,0 arc90 68.58,34.29 arc90 34.29,68.58 arc90 0,34.29 arc90
  pour Bottom: 34.29,0 arc90 68.58,34.29 arc90 34.29,68.58 arc90 0,34.29 arc90
GPIO0
  Top 0.254: U4.33 35.54,46.69 36.83,45.4 36.81,45.1 R14.2
LEFT  (via drill 0.51)
  Top 0.254: JP5.TIP 47.71,53.89 v45.72,55.88 41.91,55.88 41.26,55.23 R10.2 40.64,54.61 v39.85,53.82 U4.46 | U1.22 54.54,30.71 53.18,32.07 52.7,32.07 v51.12,33.66
  Bottom 0.254: SJ4.2 52.07,57.15 50.8,57.15 48.89,55.24 46.35,55.24 v45.72,55.88 | v39.85,53.82 50.16,43.5 50.16,34.61 v51.12,33.66
MISO  (via drill 0.51)
  Top 0.254: U7.7 16.14,22.81 v18.73,25.4 | U4.30 34.04,45.81 34.61,45.24 34.61,43.27 35.24,42.64 35.24,35.08 36.35,33.97 39.21,33.97 v40.16,33.02 | v40.16,33.02 | 45.09,31.49 44.08,31.49 42.55,33.02 v40.16,33.02 | 45.09,31.49 U1.16 | JP4.1 45.09,29.1 45.09,31.49
  Bottom 0.254: v18.73,25.4 19.05,25.72 33.97,25.72 40.16,31.91 v40.16,33.02
MOSI  (via drill 0.51)
  Top 0.254: U7.3 19.25,19.88 v21.59,22.23 | v38.73,33.02 36.35,33.02 34.61,34.77 34.61,42.35 33.97,42.99 33.97,45.09 33.54,45.52 U4.29 | U1.15 44.23,32.29 42.55,33.97 v41.27,33.97
  Bottom 0.254: JP4.4 44.08,22.17 42.86,20.95 41.59,20.95 38.1,24.45 23.81,24.45 v21.59,22.23 20,22.23 17.78,24.45 17.78,25.72 18.41,26.35 33.66,26.35 38.73,31.43 v38.73,33.02 39.69,33.97 v41.27,33.97
MP3-CS  (via drill 0.51)
  Top 0.254: U4.23 31.09,49.82 v31.75,50.48 | U1.10 50.26,36.29 50.48,36.51 50.48,37.15 46.99,40.64 v44.45,40.64
  Bottom 0.254: v31.75,50.48 29.84,50.48 27.3,47.94 27.3,46.67 29.21,44.77 38.1,44.77 39.05,45.72 41.59,45.72 44.45,42.86 v44.45,40.64
MP3-DCS  (via drill 0.51)
  Top 0.254: U4.13 29.32,54.82 28.89,55.24 v28.89,56.2 | U1.11 47.38,35.49 v46.35,36.51
  Bottom 0.254: v28.89,56.2 33.97,56.2 37.78,52.39 37.78,49.53 39.37,47.94 42.86,47.94 47.31,43.49 47.31,37.47 v46.35,36.51
MP3-DREQ  (via drill 0.51)
  Top 0.254: U4.8 33.54,57.19 34.29,57.94 v34.29,58.42 | U1.32 56.77,37.09 v55.88,36.2
  Bottom 0.254: v34.29,58.42 40.96,58.42 56.52,42.86 56.52,36.83 v55.88,36.2
MP3-MIDI-RX  (via drill 0.51)
  Top 0.254: U4.26 32.04,46.59 v31.75,46.3 31.11,45.67 R5.1
  Bottom 0.254: v31.75,46.3 32.65,45.4 33.02,45.4 37.78,45.4 38.42,46.04 38.42,46.99 35.56,49.85 35.56,50.96 36.54,51.94 36.54,52.68 34.61,54.61 25.4,54.61 20.32,49.53 20.32,47.94 13.65,41.27 13.65,36.51 13.65,20.64 15.24,19.05 18.41,15.88 SJ3.1
MP3-RST  (via drill 0.51)
  Top 0.254: v38.42,56.83 38.42,57.78 37.78,58.42 R7.2 36.84,57.96 36.04,57.15 U4.3 | U1.12 46.59,34.69 v46.35,34.92
  Bottom 0.254: v38.42,56.83 38.42,50.16 39.69,48.89 42.86,48.89 48.26,43.5 48.26,36.83 v46.35,34.92
N$1
  Top 0.254: U1.7 51.34,39.27 52.14,40.08 Y1.1
N$3
  Top 0.254: U1.8 50.54,39.31 49.74,40.11 Y1.3
N$4
  Top 0.254: U4.44 40.12,52.82 40.64,53.34 C13.2
N$5
  Top 0.254: C16.1 R12.1
N$6
  Top 0.254: R8.1 14.59,44.35 LED1.A
N$7
  Top 0.254: C15.1 R10.1
N$8
  Top 0.254: R9.2 27.32,44.35 LED2.C
N$9
  Top 0.254: U4.18 27.87,52.32 26.97,51.42 R4.2 26.02,51.42 25.4,50.8 25.4,50.34 Y2.3 25.28,48.76 C11.2
N$10
  Top 0.254: U4.17 26.98,52.82 26.88,52.72 R4.1 26.49,52.72 26.1,52.32 24.19,52.32 22.86,53.66 22.86,53.8 Y2.1 22.98,55.38 C12.2
N$11
  Top 0.254: C14.1 R11.1
N$12  (via drill 0.51)
  Top 0.254: v42.55,36.83 R24.2
  Bottom 0.254: v42.55,36.83 39.05,40.32 37.15,40.32 33.24,36.41 S2.1
N$13  (via drill 0.51)
  Top 0.254: v42.55,38.1 R25.2
  Bottom 0.254: v42.55,38.1 39.69,40.96 36.51,40.96 33.38,37.83 S2.2
N$14  (via drill 0.51)
  Top 0.254: v42.55,39.37 R26.2
  Bottom 0.254: v42.55,39.37 40.32,41.59 35.88,41.59 33.67,39.38 32.02,39.38 S2.4
N$16
  Top 0.254: 32.97,12.65 33.29,12.97 U6.6
  Top 0.406: 32.97,12.65 30.8,10.48 30.8,6.03 30.48,5.71 29.53,5.71 29.21,6.03 L1.1
N$17
  Top 0.254: U6.7 33.79,12.36 33.47,12.04
  Top 0.406: 33.47,12.04 31.59,10.16 31.59,5.71 30.8,4.92 27.78,4.92 26.67,6.03 L2.1
N$18
  Top 0.254: U6.10 35.29,12.97 35.61,12.65
  Top 0.406: 35.61,12.65 37.78,10.48 37.78,6.03 38.1,5.71 39.05,5.71 39.37,6.03 L3.1
N$19
  Top 0.254: U6.9 34.79,12.36 35.11,12.04
  Top 0.406: 35.11,12.04 36.99,10.16 36.99,5.71 37.78,4.92 40.8,4.92 41.91,6.03 L4.1
N$70
  Top 0.406: U3.4 7.65,40.02 C17.1
N$73
  Top 0.254: U4.36 37.91,47.82 39.37,46.35 R16.2
PROG
  Top 0.254: R1.1 R1X.P$1
  Top 0.406: U2.5 7.65,28.61 9.52,30.48 R1X.P$1
RIGHT  (via drill 0.51)
  Top 0.254: 41.26,49.21 R11.2 | 41.26,49.21 51.75,49.21 53.97,51.44 v55.88,51.44 56.31,51.44 JP5.RING | U1.19 52.14,31.36 v51.12,32.38 | U4.39 v39.85,50.32 39.85,49.69 40,49.53 40.32,49.21 41.26,49.21
  Bottom 0.254: SJ5.2 55.88,52.7 v55.88,51.44 | v51.12,32.38 49.21,34.29 49.21,43.5 42.39,50.32 v39.85,50.32
ROT-A  (via drill 0.51)
  Top 0.254: C24.1 38.91,26.13 S2.A | U1.1 56.14,40.06 v55.56,40.64
  Bottom 0.254: S2.A 40.24,27.22 43.34,30.16 54.77,30.16 55.88,31.27 55.88,33.5 54.93,34.45 54.93,40 v55.56,40.64
ROT-B  (via drill 0.51)
  Top 0.254: C25.1 42.45,29.67 S2.B | U1.26 57.62,32.31 v55.01,32.31
  Bottom 0.254: S2.B 53.46,30.75 v55.01,32.31
ROT-LEDB
  Top 0.254: U1.9 48.63,37.09 46.35,39.37 R26.1
ROT-LEDG  (via drill 0.51)
  Top 0.254: U1.24 56.14,28.2 54.93,26.99 48.58,26.99 42.86,21.27 41.59,21.27 34.92,27.94 34.92,29.84 31.59,33.18 31.59,38.89 v33.02,40.32 | v46.35,38.1 R25.1
  Bottom 0.254: v33.02,40.32 34.92,42.23 40.96,42.23 45.09,38.1 v46.35,38.1
ROT-LEDR
  Top 0.254: U1.14 44.38,33.09 42.86,34.61 42.86,35.24 43.5,35.88 44.77,35.88 45.1,36.21 R24.1
ROT-SW  (via drill 0.51)
  Top 0.254: R2.2 57.77,41.91 v55.56,41.91 54.77,41.12 54.77,40.16 55.34,39.59 U1.2
  Bottom 0.254: S2.3 26.54,39.24 24.61,37.31 24.61,35.4 25.72,34.29 34.61,34.29 36.2,35.88 44.13,35.88 48.58,31.43 53.02,31.43 53.97,32.38 53.97,40.32 v55.56,41.91
RST  (via drill 0.51)
  Top 0.254: R3.1 C4.2 57.78,38.73 56.52,37.46 55.56,37.46 54.93,36.83 54.93,35.88 v55.88,34.92 56.11,34.69 U1.29
  Bottom 0.254: JP4.5 42.28,24.5 47.31,29.53 54.93,29.53 56.52,31.11 56.52,34.29 v55.88,34.92
SCK  (via drill 0.51)
  Top 0.254: U7.5 17.69,21.19 v20.32,23.81 | U1.17 50.54,28.99 49.8,28.26 46.04,28.26 44.08,26.3 JP4.3 42.28,28.15 43.81,29.69 43.81,30.8 42.55,32.07 36.35,32.07 33.97,34.45 33.97,42.07 33.34,42.7 33.34,44.93 33.04,45.22 U4.28
  Bottom 0.254: JP4.3 39.63,26.3 38.42,25.08 21.59,25.08 v20.32,23.81
SD-CS  (via drill 0.51)
  Top 0.254: U7.2 20.38,19.11 v22.54,21.27 | U1.13 44.85,33.89 v43.81,34.92
  Bottom 0.254: v22.54,21.27 19.68,21.27 16.77,24.18 16.77,25.98 17.78,26.99 33.34,26.99 37.78,31.43 37.78,33.34 39.37,34.92 v43.81,34.92
SPKL+
  Top 0.406: L3.2 TP7.1 39.37,10.48 40,11.11 C32.1
  Bottom 0.406: TP7.1 35.56,10.16 34.29,8.89 ST6.1
SPKL-
  Top 0.406: C33.1 41.27,11.11 41.91,10.48 TP6.1 L4.2
  Bottom 0.406: ST5.1 49.62,7.62 44.45,7.62 TP6.1
SPKR+
  Top 0.406: L1.2 TP9.1 29.21,10.48 28.57,11.11 C30.1
  Bottom 0.406: TP9.1 27.62,11.75 21.27,11.75 11.75,21.27 ST8.1
SPKR-
  Top 0.406: L2.2 TP8.1 26.67,10.48 27.3,11.11 C31.1
  Bottom 0.406: ST7.1 18.96,7.62 24.13,7.62 TP8.1
STAT
  Top 0.254: U2.1 4.12,27.62 3.81,27.3 3.81,24.45 5.08,23.18 12.06,23.18 20.95,32.07 23.18,32.07 23.97,32.86 23.97,38.58 26.02,40.62 R9.1
TRIG1  (via drill 0.51)
  Top 0.254: U1.23 55.34,30.7 v53.02,33.02
  Bottom 0.254: v53.02,33.02 51.12,34.92 51.12,43.81 39.37,55.56 39.37,57.15 38.73,57.78 34.92,57.78 34.61,57.47 33.97,57.47 33.34,58.1 33.34,59.37 TP1.1 ST12.1
TRIG2/SDA  (via drill 0.51)
  Top 0.254: U1.27 55.49,33.09 55.24,33.34 54.61,33.34 v53.02,34.92 | v36.67,34.92 37.62,35.88 39.69,35.88 40.64,36.83 40.64,42.55 42.86,44.77 47.94,44.77 v50.48,47.31 | U6.19 33.79,20.66 33.5,20.95 29.84,20.95 25.4,20.95 24.77,20.32 24.77,15.88 24.77,14.61 | v20,28.89 24.13,24.77 24.13,17.14 22.23,15.24 18.41,15.24 17.78,15.24 SJ2.2 SJ2.1 18.42,14.61 20.32,14.61 23.49,14.61 24.77,14.61 | v40.64,57.15 46.99,57.15 TP2.1 | R18.2 24.77,14.61
  Bottom 0.254: v53.02,34.92 52.07,35.88 52.07,44.29 50.48,45.88 v50.48,47.31 v40.64,57.15 | TP2.1 ST1.1 | v20,28.89 20.64,28.26 32.7,28.26 36.2,31.75 36.2,34.45 v36.67,34.92
TRIG3/SCL  (via drill 0.51)
  Top 0.254: U1.28 55.33,33.89 v53.02,36.2 | v38.1,34.92 40,34.92 41.27,36.2 41.27,42.39 43.02,44.13 50.48,44.13 v52.07,45.72 53.66,47.31 TP3.1 | U6.17 34.79,21.14 v35.56,21.91 | v23.18,17.46 21.59,15.88 17.46,15.88 15.72,17.62 15.08,17.62 SJ1.1 SJ1.2 14.45,18.26 16.03,18.26 17.78,16.51 20.8,16.51 23.49,19.21 23.49,23.49 v19.05,27.94 | R19.2 v26.03,14.61
  Bottom 0.254: TP3.1 ST2.1 | v53.02,36.2 53.02,44.77 v52.07,45.72 | v38.1,34.92 36.99,33.81 36.99,31.59 33.02,27.62 19.37,27.62 v19.05,27.94 | v35.56,21.91 34.61,22.86 27.15,22.86 23.18,18.89 v23.18,17.46 v26.03,14.61
TRIG4/TXO  (via drill 0.51)
  Top 0.254: U1.31 59.59,36.29 60.33,35.56 TP4.1 60.33,27.62 48.58,15.88 47.94,15.24 | 47.94,15.24 46.35,13.65 v45.4,13.65 | JP2.2 47.94,15.25 47.94,15.24
  Bottom 0.254: TP4.1 ST3.1 | SJ3.2 19.05,15.24 21.59,12.7 44.13,12.7 44.45,12.7 v45.4,13.65
TRIG5/RXI  (via drill 0.51)
  Top 0.254: U1.30 58.65,35.49 58.9,35.25 58.9,33.66 59.69,32.86 59.69,27.94 56.2,24.45 v55.56,24.45 55.56,23.81 48.89,17.14 47.98,17.14 R22.1
  Bottom 0.254: TP5.1 60.96,18.96 ST4.1 55.56,22.23 v55.56,24.45
VBATT  (via drill 0.51)
  Top 0.406: JP1.2 16.3,53.97 JP3.2 | U2.3 5.05,24.8 5.71,24.13 v8.89,24.13 9.51,24.75 C10.1 | v12.7,38.73 16.12,38.73 S1.1
  Bottom 0.406: JP3.2 18.94,48.47 12.7,42.23 v12.7,38.73 12.7,28.57 12.7,25.72 11.11,24.13 v8.89,24.13
VBATT_SW  (via drill 0.51)
  Top 0.254: U6.4 31.59,17.28 31.59,16.78 | U6.5 31.59,16.78 | U6.11 37.15,16.78 | U6.13 37.31,17.78 37.78,17.3 37.78,14.84 v37.46,14.61 37.15,14.84 37.15,16.78 | 31.59,16.78 v31.59,14.61 | U6.12 37.15,17.28 37.15,16.78 | C23.1 30.04,27.15 30.32,27.15
  Top 0.406: U3.1 3.81,42.86 | 3.81,42.86 3.81,42.55 3.81,40.96 | 3.81,40.96 3.81,39.05 5.71,37.15 7.94,37.15 9.52,35.56 13.97,35.56 15.24,34.29 v16.51,34.29 S1.2 20.98,37.21 C2.A | U3.3 3.81,40.96 | v33.02,21.91 33.02,23.36 C22.A 32.89,24.58 30.32,27.15 v28.26,29.21 | D1.C 4.68,45.32 3.81,44.45 3.81,43.17 3.81,42.86
  Bottom 0.406: v37.46,14.61 v31.59,14.61 30.32,13.34 28.26,13.34 27.46,14.13 27.46,18.89 30.48,21.91 v33.02,21.91 | v16.51,34.29 21.59,29.21 v28.26,29.21
VIN  (via drill 0.51)
  Top 0.254: LED2.A 25.08,43.61 25.08,40.64 23.34,38.89 23.34,33.18 22.86,32.7 20.64,32.7 18.1,30.16 16.03,30.16 15.24,29.37 v15.24,28.57 | 7.94,25.72 U2.4
  Top 0.406: JP2.4 v47.67,22.7 | 7.94,25.72 8.57,26.35 8.57,26.99 8.89,27.3 C9.1 9.51,28.24 9.84,28.57 v11.75,28.57 v15.24,28.57
  Bottom 0.406: v15.24,28.57 15.24,24.13 19.37,20 23.18,20 26.83,23.65 37.78,23.65 41.27,20.16 45.13,20.16 v47.67,22.7 | v11.75,28.57 TP11.1 ST10.1

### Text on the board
Bottom: V15
tPlace: T1 | GND | SDA | T2 | 3.5-6V | + | VIN | - | Power | Charge | T3 | SCL | ON | T4 | TXO | R1 | 3.3V | OFF | BLK | ISP | T5 | RXI | + | SJ1 | SPEAKER | RIGHT | SJ2 | - | GRN | 5V FTDI | MP3 | - | LEFT | + | SPEAKER
bPlace: T1 | GND | SDA | T2 | SJ4 | 3.7-6V | SJ5 | VIN | VBATT | GND | T3 | SCL | LilyPad MP3 | 1.8V | 3.3V | T4 | TXO | SJ3 | T5 | + | DTR | RXI | -L+ | +R- | RIGHT | - | SPEAKER | - | LEFT | SPEAKER | +
tValues: N. Seidle, M. Grusin

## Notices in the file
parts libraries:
SparkFun: Released under the Creative Commons Attribution Share-Alike 3.0 License
SparkFun: http://creativecommons.org/licenses/by-sa/3.0
SparkFun-Passives: Licensing: CC v3.0 Share-Alike You are welcome to use this library for commercial purposes.
